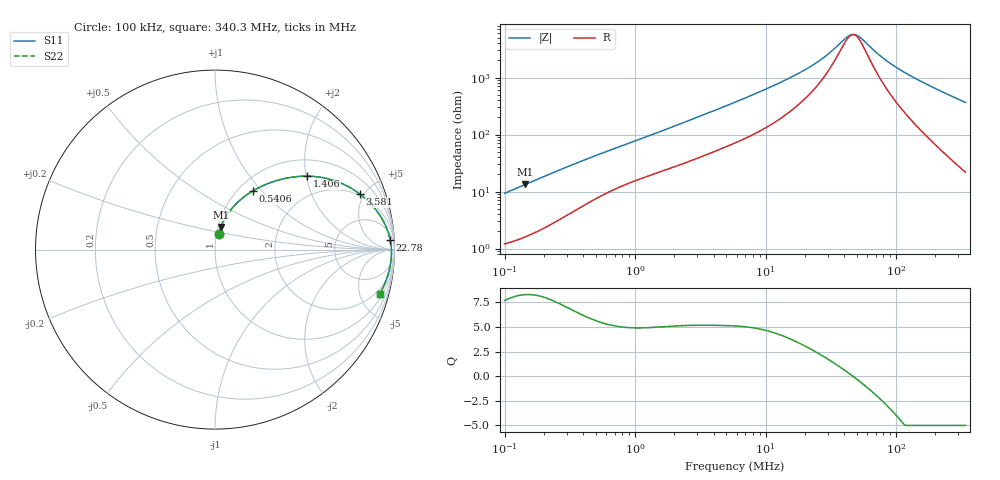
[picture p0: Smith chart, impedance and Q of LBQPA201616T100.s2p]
! LBQPA201616T100  S-PARAMETER MODEL  ( General Type )
! Model Generated by TAIYO YUDEN Corporation (http://www.ty-top.com)
! Version 1.0
! TAIYO YUDEN Control No. 191025NI43SB-FBB
! Copyright(c) 2019 TAIYO YUDEN CO.,LTD. All Rights Reserved.
! Product Description (link to TY-COMPAS)
! https://ds.yuden.co.jp/TYCOMPAS/or/detail?pn=LBQPA201616T100K&u=M
! Products Name : Inductors
! Characteristics :
!  Inductance : 10 uH , SRF(min) : 32 MHz , DC Resistance(max) : 1.066 Ohm
!  Rated Current : Saturation :380 mA , Temp Rise : 305 mA (20 degC)
!  Case Size : 2.0 x 1.6 / 0.079 x 0.063 [mm/inch] , Thickness : 1.6 / 0.063 [mm/inch]
!  (Conditions: Temperature = 25 degC , DC Bias Current/Voltage = 0A / 0V)
! External Node Assignments :
!  1  o---GGG---o  2
! GND o---------o GND
! Frequency Range : 0.1MHz  -  340.31115MHz  [ 402 STEP ]
# MHz S RI R 50
! Freq[MHz].  S11 Real  S11 Imag  S21 Real  S21 Imag  S12 Real  S12 Imag  S22 Real  S22 Imag
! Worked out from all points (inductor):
!   401 points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, 100 kHz to 340.3 MHz, reference 50 ohm
!   read as one part in series: L = 14.7 uH near 104.2 kHz
!   highest Q = 8.28 at 144.2 kHz (marker M1), where L = 14.6 uH
!   self-resonance near 46.7 MHz
!   S11 on the Smith chart (normalised r, x): 100 kHz: 1.02, +0.18; 540.6 kHz: 1.16, +0.90; 1.406 MHz: 1.41, +2.03; 3.581 MHz: 1.90, +4.65; 22.78 MHz: 12, +31; 340.3 MHz: 1.44, -7.31
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0.1  0.0201 0.0895  0.9799 -0.0895  0.9799 -0.0895  0.0201 0.0895
0.14419  0.0322 0.1263  0.9678 -0.1263  0.9678 -0.1263  0.0322 0.1263
0.244628  0.071 0.1991  0.929 -0.1991  0.929 -0.1991  0.071 0.1991
0.390471  0.1406 0.2765  0.8594 -0.2765  0.8594 -0.2765  0.1406 0.2765
0.540585  0.2127 0.328  0.7873 -0.328  0.7873 -0.328  0.2127 0.328
0.917141  0.3657 0.3906  0.6343 -0.3906  0.6343 -0.3906  0.3657 0.3906
1.405594  0.5137 0.4091  0.4863 -0.4091  0.4863 -0.4091  0.5137 0.4091
1.524679  0.543 0.4079  0.457 -0.4079  0.457 -0.4079  0.543 0.4079
2.243586  0.6773 0.3801  0.3227 -0.3801  0.3227 -0.3801  0.6773 0.3801
3.581175  0.8069 0.3097  0.1931 -0.3097  0.1931 -0.3097  0.8069 0.3097
5.953437  0.8965 0.2219  0.1035 -0.2219  0.1035 -0.2219  0.8965 0.2219
12.89128  0.9595 0.1114  0.0405 -0.1114  0.0405 -0.1114  0.9595 0.1114
22.77862  0.9759 0.0548  0.0241 -0.0548  0.0241 -0.0548  0.9759 0.0548
30.2791  0.9799 0.0319  0.0201 -0.0319  0.0201 -0.0319  0.9799 0.0319
41.91969  0.9824 0.00784  0.0176 -0.00784  0.0176 -0.00784  0.9824 0.00784
47.35831  0.9829 -0.00101  0.0171 0.00101  0.0171 0.00101  0.9829 -0.00101
53.50253  0.9831 -0.00994  0.0169 0.00994  0.0169 0.00994  0.9831 -0.00994
71.11972  0.9827 -0.0317  0.0173 0.0317  0.0173 0.0317  0.9827 -0.0317
88.94399  0.9814 -0.0506  0.0186 0.0506  0.0186 0.0506  0.9814 -0.0506
115.8517  0.9783 -0.0761  0.0217 0.0761  0.0217 0.0761  0.9783 -0.0761
157.1621  0.9715 -0.1117  0.0285 0.1117  0.0285 0.1117  0.9715 -0.1117
340.3111  0.918 -0.2462  0.082 0.2462  0.082 0.2462  0.918 -0.2462
